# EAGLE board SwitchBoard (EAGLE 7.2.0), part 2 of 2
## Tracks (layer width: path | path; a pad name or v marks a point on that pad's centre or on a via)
5VIN  (via drill 0.4)
  Top 0.254: LED1.A 0.63,71.53 0.63,71.12 0.82,70.93 0.89,70.87 1.02,70.74 4.95,70.74 v5.08,70.87
  Top 0.406: X1.VBUS 6.32,78.77 JP1.1 8.57,78.74 C1.1 U1.4 | 0.63,71.53 LED1.A
  Bottom 0.406: 7.3,73.98 6.98,73.66 6.35,73.03 | 7.3,73.98 8.25,74.93 8.25,77.47 7.62,78.1 | 7.62,78.1 | 7.62,78.1 6.98,78.74 JP1.1 | v5.08,70.87 5.46,70.87 5.71,71.12 5.71,72.39 7.3,73.98
+5V  (via drill 0.6)
  Top 0.406: C21.1 C20.1 13.65,62.87 12.7,62.87 12.06,62.23 12.06,58.42 11.43,57.78 6.98,57.78 6.35,57.15 X2.9 | C21.1 | U12.1 18.41,62.23 17.46,63.18 C21.1 | U15.1 | U15.1 18.41,48.26 17.46,49.21 C26.1 C27.1 12.38,49.21 v12.06,49.53 | X2.9
  Bottom 0.406: v12.06,49.53 12.06,53.98 11.75,54.29 | 11.75,54.29 11.43,54.61 | 11.12,54.91 11.43,54.61 | 11.43,54.61 11.75,54.29 | X2.9 11.12,54.91 | 11.12,54.91 11.43,54.61
AGND  (via drill 0.4, 0.5, 0.6)
  Top 0.254: U12.9 U12.10 | U4.EXP v30.61,79.5 | 29.52,78.41 v29.08,77.98 | C15.- 41.31,86.96 U8.EXP 41.27,87.63 40.66,88.25 U8.7 | LED2.C 0.86,69.94 1.08,70.17 4.13,70.17 4.45,69.85 5.71,69.85 6.35,70.49 v6.98,70.49
  Top 0.406: v59.05,32.38 59.33,32.11 U5.21 | v55.88,29.21 55.88,28.58 55.88,27.94 57.15,26.67 57.78,26.67 58.42,26.04 59.05,25.4 59.33,25.12 U5.4 59.33,17.82 C7.1 59.05,17.46 v59.05,15.88 59.05,8.89 59.05,8.25 64.14,3.17 65.41,3.17 | v64.14,79.38 64.14,76.84 59.69,72.39 59.69,67.03 59.33,66.68 59.33,64.41 v59.05,64.13 59.33,63.85 U2.21 59.33,58.77 59.33,55.52 U2.4 59.37,54.3 C8.1 60,50.16 61.59,50.16 v62.23,49.53 | U7.4 141.96,22.58 v142.24,22.86 142.56,23.18 C13.1 | C17.1 142.56,51.12 v142.24,50.8 141.96,50.52 141.96,49.89 U10.4 141.96,46.71 141.96,44.73 U10.21 141.96,39.01 v141.96,38.38 141.96,34.92 143.51,33.38 143.51,30.48 144.15,29.84 148.59,29.84 156.21,37.46 156.21,45.72 157.48,46.99 157.81,47.32 160.35,47.32 X3.6 164.77,47.32 165.74,46.35 165.74,35.56 163.83,33.66 | U13.4 141.96,75.92 v142.24,76.2 142.24,77.78 C23.1 | U13.21 U13.20 U13.19 140.67,69.55 v141.6,70.49 | U13.16 U13.15 138.05,67.06 v138.43,66.68 | v141.6,16.51 141.96,16.15 U7.21 141.96,10.16 141.96,7.98 137.16,3.17 136.53,3.17 134.34,3.17 133.99,3.17 130.81,3.17 66.04,3.17 65.41,3.17 | U15.15 31.43,46.99 C24.2 C25.2 34.61,46.99 35.25,47.62 v36.2,47.62 | 27.94,46.99 27.3,46.35 27.3,41.27 27.94,40.64 U15.10 U15.9 | 27.94,46.99 U15.15 | U15.15 | U12.10 27.94,54.61 27.3,55.24 27.3,60.32 27.94,60.96 | 27.94,60.96 U12.15 31.43,60.96 C19.2 C18.2 35.25,61.28 35.56,61.28 v35.88,61.28 | U15.15 27.94,46.99 | 27.94,46.99 27.3,47.62 27.3,52.7 27.94,53.34 U12.9 | 163.83,33.66 | 163.83,33.66 JP5.1 | X1.GND 6.32,76.17 JP1.2 8.57,76.2 C1.2 8.89,75.56 9.52,74.93 9.52,73.66 10.16,73.03 12.7,73.03 13.02,73.34
  Top 0.406: U15.9 32.38,39.37 33.34,39.37 R24.1 | U4.7 U4.6 | U4.6 U4.5 | U4.6 28.17,78.74 U4.EXP | U4.EXP v30.61,77.98 30.82,77.76 U4.13 32.09,77.76 32.38,77.47 32.38,76.84 33.02,76.2 33.97,76.2 R10.1 33.97,75.56 R5.1 | U4.10 29.52,78.41 U4.EXP | C3.2 C4.2 24.45,78.74 | R11.2 2.22,87.95 1.9,87.63 1.49,87.22 0.86,86.58 LED4.C 0.86,83.6 1.27,83.19 1.9,83.19 3.17,83.19 v4.45,81.28 8.89,81.28 9.52,81.28 10.16,81.91 10.79,82.55 JP2.2 | JP2.2 10.79,84.29 JP3.1 | 13.02,73.34 R3.1 13.02,73.34 | U1.2 14.92,77.47 C2.2 | C9.2 C11.2 37.47,84.46 39.37,82.55 C15.- 39.37,80.6 39.37,79.38 | 27.94,60.96 27.3,61.6 27.3,62.87 33.97,69.53 R5.1 | 39.37,79.34 39.37,79.38 | 65.41,3.17 64.77,3.17 | R23.1 37.15,42.55 v35.56,42.55 | U15.9 29.46,40.01 v30.48,40.01 30.48,33.66 25.4,28.58 JP6.2 | 39.37,79.38 39.37,76.84 36.2,73.66 R5.1 | 13.33,95.25 10.79,92.71 JP2.2
  Bottom 0.254: v6.98,70.49 8.25,70.49 8.89,71.12 8.89,73.66 9.52,74.29 9.52,79.38 7.62,81.28 v4.45,81.28
  Bottom 0.406: v59.05,64.13 59.33,64.41 U3.21 59.33,70.49 | 59.33,70.49 59.33,70.76 | C6.1 59.33,79.97 U3.4 59.33,72.75 59.33,70.49 | v55.88,29.21 v59.05,32.38 59.33,32.66 U6.21 59.33,37.74 59.33,39.02 59.33,39.73 v59.05,40.01 59.33,40.28 U6.4 59.33,46 59.69,46.35 60.33,46.99 60.96,46.99 | 60.96,82.55 62.86,80.65 63.5,80.01 v64.14,79.38 | C17.1 142.88,52.39 142.88,51.44 v142.24,50.8 141.96,51.08 U11.4 141.96,58.06 141.96,60.04 U11.21 141.96,65.69 141.6,66.04 | v142.24,76.2 142.24,77.78 C23.1 | 142.08,78.58 141.96,78.71 U14.4 141.96,84.74 140.97,85.72 140.34,86.36 | 142.08,78.58 C23.1 | v141.96,38.38 141.96,37.19 U9.21 141.96,32.1 141.96,30.12 U9.4 141.96,27.59 141.96,25.37 C13.1 142.24,24.45 v142.24,22.86 140.97,21.59 140.97,17.14 v141.6,16.51 | U14.15 U14.16 138.71,86.72 139.06,86.36 140.34,86.36 | 140.34,86.36 140.66,86.69 U14.19 U14.20 U14.21 | 141.6,66.04 139.7,66.04 139.06,66.04 v138.43,66.68 | 141.6,66.04 v141.6,70.49 140.34,71.75 140.34,73.66 140.34,76.84 142.08,78.58 | v4.45,81.28 4.45,78.1 JP1.2 | v30.48,40.01 33.02,42.55 34.92,42.55 v35.56,42.55 35.56,46.35 36.2,46.99 v36.2,47.62 | C23.1 | C23.1 | 60.96,46.99 61.59,46.99 62.23,47.62 v62.23,49.53 | C8.1 59.37,48.58 60.96,46.99 | v35.88,61.28 37.14,61.28 40.64,57.78 40.64,53.98 40.64,52.7 41.27,52.07 JP7.3 | JP7.3
  other vias: 29.08,79.5 29.84,78.74 26.04,81.91 41.27,89.53 41.27,84.46 19.05,95.25 46.99,87 48.26,85.72 48.89,83.82 48.89,80.01 48.89,78.1 27.3,80.01 26.04,78.74 156.84,45.72 155.58,48.9 153.03,45.72 151.13,52.7 151.13,55.88 50.17,65.41 55.25,69.22 52.39,80.96 50.8,83.19 52.7,83.19 71.12,17.78 71.12,12.7 71.12,5.08 46.99,80.01 45.09,80.01 33.66,89.53 31.75,89.53 31.75,91.44 31.75,93.34 31.75,95.25 19.05,93.34 19.05,91.44 19.05,89.53 38.1,81.28 36.83,81.28 34.92,82.55 71.12,15.24 68.58,17.78 65.41,17.78 62.23,17.78 71.12,46.99 71.12,49.53 67.31,49.53 67.31,46.99 64.14,46.99 64.14,49.53 66.67,79.38 68.58,79.38 71.12,79.38 71.12,81.28 71.12,83.19 71.12,85.09 133.35,67.31 130.81,67.31 130.81,70.49 133.35,70.49 133.35,73.66 130.81,73.66 133.35,81.28 130.81,81.28 130.81,83.82 133.35,83.82 130.81,5.08 136.53,10.16 138.43,10.16 142.88,10.16 20.32,85.09 20.32,83.19 19.05,81.91 71.12,93.34 71.12,96.52 130.81,95.88 1.27,30.48 1.27,1.27 27.81,51.69 30.48,54.74 33.02,54.74 33.15,51.18 29.59,50.93 27.81,49.91 28.7,38.1 27.56,36.07 26.42,34.29
  pour Top (no thermals): 27.3,55.24 32.38,55.24 32.38,52.7 27.3,52.7
  pour Top (no thermals): 27.3,41.27 31.75,41.27 31.75,38.73 27.3,38.73
  pour Top (isolate 0.305, no thermals): 40.64,85.72 40.64,83.19 41.91,83.19 41.91,85.72
  pour Top (no thermals): 41.91,88.26 41.91,90.17 40.64,90.17 40.64,88.26
  pour Top (no thermals): 26.42,78.3 28.96,78.3 28.96,79.88 28.26,79.88 28.26,81.03 27.3,81.91 27.3,87 24.13,87 24.13,82.55 25.4,82.55 25.4,79.38 20.95,79.38 20.95,78.1 26.04,78.1
  pour Bottom (isolate 0.305, no thermals): 20.32,69.22 20.32,87 38.73,87 38.73,69.22
  pour Top (isolate 0.305, no thermals): 37.47,85.09 41.27,85.09 41.27,82.55 38.73,82.55 37.47,83.82
  pour Bottom (isolate 0.305, rank 6): -3.81,67.94 -3.81,102.87 -3.18,103.5 172.09,103.5 172.09,-2.54 -3.81,-2.54 -4.45,-1.91 -4.45,33.02 -3.18,33.02 -0.64,32.38 22.23,32.38 22.86,33.02 22.86,34.29 26.04,37.46 26.04,63.5 25.4,64.13 24.13,67.94
  pour Top (isolate 0.305, rank 6): -7.62,32.38 -11.43,-3.81 175.26,-3.81 173.99,104.78 -8.25,105.41 -6.35,67.94 24.13,67.94 26.04,63.5 26.04,38.1 22.23,32.38
CHRG
  Top 0.406: R1.2 LED1.C
DIN+  (via drill 0.6)
  Top 0.406: U2.3 58.67,56.26 56.52,58.42 55.88,58.42 55.25,57.78 55.25,55.24 v54.61,54.61 | U12.13 v36.83,58.42 37.47,59.05 48.26,59.05 49.53,59.05 | 49.53,59.05 v50.17,59.69 49.53,59.05
  Bottom 0.406: v36.83,58.42 37.47,58.42 39.37,56.52 39.37,48.9 41.27,46.99 JP7.7 | JP7.7 | JP7.7 | v54.61,54.61 53.97,54.61 53.34,55.24 53.34,55.88 53.97,56.52 53.97,57.78 53.34,58.42 51.44,58.42 v50.17,59.69
DIN+2  (via drill 0.5)
  Top 0.406: U2.22 58.67,58.67 v58.42,58.42 | v53.97,49.53 53.97,46.99 53.34,46.35 53.34,33.02 v53.97,32.38 | U5.3 58.67,24.51 57.78,25.4 v57.15,25.4
  Bottom 0.406: v57.15,25.4 55.88,26.67 53.97,28.58 v53.97,32.38 | v53.97,49.53 53.97,50.8 55.25,52.07 57.15,53.98 | v58.42,58.42 58.42,55.24 57.15,53.98 | 57.15,53.98 55.25,55.88 55.25,57.47 55.25,58.74 R6.1
DIN+3  (via drill 0.5)
  Top 0.406: U5.22 58.67,27.05 v60.33,25.4 | U7.3 142.62,19.43 v142.24,19.05
  Bottom 0.406: v60.33,25.4 60.33,24.13 | R12.1 55.56,22.54 57.15,24.13 60.33,24.13 | 67.94,2.54 78.11,2.54 130.81,2.54 131.44,2.54 132.08,2.54 138.43,2.54 140.97,5.08 140.97,11.43 140.97,13.97 142.88,15.88 142.88,16.51 142.88,17.78 142.24,18.41 v142.24,19.05 | 67.94,2.54 67.31,2.54 | 60.33,24.13 60.33,20.95 60.33,6.98 63.5,3.81 64.77,2.54 67.94,2.54
DIN+4  (via drill 0.5)
  Top 0.406: U7.22 142.62,12.32 143.19,11.75 R17.1 149.54,11.75 150.18,11.75 v151.13,12.7 | U10.3 142.62,46.61 142.88,46.35 143.51,46.35 146.05,46.35 146.69,45.72 v146.69,43.81
  Bottom 0.406: v151.13,12.7 151.13,41.91 149.86,43.18 147.96,43.18 147.32,43.18 v146.69,43.81
DIN+5
  Top 0.406: 147.63,39.37 R19.1 | R19.1 150.18,39.69 151.13,40.64 151.77,41.27 151.77,46.35 152.4,46.99 152.4,71.12 151.77,71.75 151.13,72.39 150.5,73.03 149.86,73.03 142.88,73.03 142.62,73.28 U13.3 | U10.22 142.62,44.2 142.88,44.45 144.15,44.45 144.78,43.81 144.78,43.18 146.05,41.91 146.05,40.64 146.69,40.01 147.64,40.01 R19.1
DIN+_DCHN  (via drill 0.6)
  Top 0.406: JP7.8 45.09,47.62 v47.62,47.62
  Bottom 0.406: X6.3 10.16,15.88 | v47.62,47.62 47.62,46.35 47.62,45.72 47.62,42.55 47.62,41.91 48.26,41.27 48.26,29.21 48.26,28.58 47.62,27.94 36.83,27.94 36.2,27.94 27.94,19.68 15.88,19.68 12.06,15.88 X6.3 | X6.3
DIN+_IN
  Top 0.406: U12.4 16.51,58.42 X2.3
DIN-  (via drill 0.5, 0.6)
  Top 0.406: U12.12 v35.56,57.15 37.47,57.15 38.42,58.1 | 38.42,58.1 38.73,58.42 | v53.34,76.2 52.7,75.56 52.7,73.66 52.07,73.03 50.17,73.03 49.53,72.39 49.53,70.49 49.53,69.85 50.17,69.22 51.44,67.94 51.44,59.05 50.8,58.42 38.73,58.42 | 38.73,58.42 38.42,58.1
  Bottom 0.406: U3.3 58.67,73.28 58.42,73.03 57.15,73.03 56.52,73.66 56.52,75.56 55.88,76.2 v53.34,76.2 | v35.56,57.15 37.47,57.15 38.73,55.88 38.73,50.8 38.73,48.26 41.91,45.09 JP7.9 | JP7.9
DIN-2  (via drill 0.5, 0.6)
  Top 0.406: v60.96,48.9 60.96,48.26 60.33,47.62 59.05,47.62 v58.42,47.62
  Bottom 0.406: 54.93,72.39 R7.1 54.92,72.71 55.25,72.39 58.42,72.39 58.67,72.14 U3.22 58.67,65.66 57.78,64.77 57.78,62.23 60.96,59.05 v60.96,48.9 | U6.3 58.67,45.09 58.67,47.37 v58.42,47.62
DIN-3  (via drill 0.5)
  Top 0.406: v51.44,38.1 51.44,20.95 51.44,20.32 53.97,17.78 53.97,8.25 61.59,0.63 62.23,0.63 64.77,0.63 134.62,0.63 142.88,0.63 | v148.59,13.97 151.77,13.97 152.4,13.34 152.4,8.89 144.15,0.63 142.88,0.63 | 143.51,0.63 142.88,0.63
  Bottom 0.406: U6.22 58.67,38.48 58.42,38.73 58.1,39.05 55.56,39.05 R13.1 52.39,39.05 v51.44,38.1 | U9.3 142.62,29.59 142.62,31.5 143.51,32.38 144.15,32.38 147.32,32.38 147.96,31.75 147.96,30.48 147.96,22.86 147.32,22.23 147.32,15.88 147.32,15.24 v148.59,13.97
DIN-4
  Bottom 0.406: U9.22 142.62,35.94 142.62,37.21 142.88,37.46 147.64,37.46 R18.1 147.96,39.37 146.69,40.64 145.42,41.91 144.78,42.55 144.15,43.18 144.15,45.72 148.59,50.16 148.59,50.8 148.59,53.98 148.59,56.52 147.32,57.78 146.05,59.05 142.88,59.05 142.62,58.8 142.62,57.53 U11.3
DIN-5
  Bottom 0.406: U14.3 142.62,83.57 142.88,83.82 144.78,83.82 148.59,80.01 148.59,76.2 147.96,75.56 | U11.22 142.62,63.88 142.88,64.13 146.05,64.13 146.69,64.77 147.64,64.77 R20.1 149.55,65.09 149.86,65.41 149.86,67.94 147.96,69.85 147.96,71.75 147.96,75.56 | 147.96,75.56
DIN-_DCHN  (via drill 0.6)
  Top 0.406: X6.7 11.43,14.5 12.06,15.14 v12.06,20.95
  Bottom 0.406: JP7.10 45.09,44.45 45.72,43.81 45.72,40.64 45.72,40.01 46.36,39.37 46.36,31.75 46.36,31.12 46.36,30.48 45.72,29.84 34.29,29.84 33.66,29.21 26.04,21.59 12.7,21.59 v12.06,20.95 | JP7.10
DIN-_IN
  Top 0.406: U12.5 16.51,57.15 10.16,50.8 10.16,49.53 10.06,49.43 X2.7
DOUT+  (via drill 0.6)
  Top 0.406: 147.64,66.68 R21.1 | U13.22 142.62,67.56 142.88,67.31 144.15,67.31 144.78,67.94 146.69,67.94 147.64,66.99 R21.1 | R21.1 147.96,62.23 v148.59,61.6 | X3.3 160.02,51.44 | 160.02,51.44 159.39,51.44 | v156.84,57.15 158.12,57.15 158.75,56.52 158.75,52.7 158.75,52.07 159.39,51.44 | 159.39,51.44 160.02,51.44
  Bottom 0.406: v148.59,61.6 151.13,61.6 155.58,57.15 v156.84,57.15
DOUT-  (via drill 0.6)
  Top 0.406: 154.31,62.87 154.31,52.7 156.95,50.06 X3.7 | 154.31,62.87 v154.31,64.13 154.31,62.87
  Bottom 0.406: 142.62,88.9 U14.22 142.62,88.9 | v154.31,64.13 153.03,65.41 153.03,69.85 151.77,71.12 151.77,80.65 146.05,86.36 R22.1 145.09,88.59 144.78,88.9 144.15,89.53 143.26,89.53 142.62,88.9
GND  (via drill 0.4)
  Top 0.406: C20.2 C21.2 16.51,60.96 U12.2 20.32,60.96 20.95,60.32 20.95,55.24 20.32,54.61 U12.7 | C20.2 | U12.8 20.32,53.34 20.95,52.7 20.95,47.62 20.32,46.99 | 20.32,46.99 20.95,46.35 20.95,41.27 20.32,40.64 U15.7 U15.8 | 20.32,46.99 | 20.32,46.99 U15.2 16.83,46.99 C26.2 C27.2 13.65,47.62 12.06,47.62 11.75,47.31 11.13,46.69 X2.6
  other vias: 19.56,65.66 0.89,65.79 18.8,50.93 20.7,50.93 18.54,35.94 0.89,35.81
  pour Top (no thermals): 20.95,55.24 20.95,52.7 15.88,52.7 15.88,55.24
  pour Top (no thermals): 20.95,41.27 20.95,38.73 15.88,38.73 15.88,41.27
  pour Top: -5.71,67.31 20.95,67.31 22.86,63.5 22.86,38.73 19.68,34.29 -6.35,34.29
  pour Bottom (isolate 0.305): -4.45,67.31 21.59,67.31 24.13,62.23 23.49,38.73 20.32,33.66 -3.81,33.66 -4.45,65.41
GND_DCHN
  Top 0.406: X6.6 13.66,11.76 14.61,12.7 14.61,20.95 15.24,21.59 26.04,21.59 34.29,29.84 45.72,29.84 46.36,30.48 46.36,44.45 46.36,45.09 45.72,45.72 43.81,45.72 43.18,46.35 43.18,51.44 43.81,52.07 JP7.4
IN+  (via drill 0.5, 0.6)
  Top 0.406: U2.19 60.63,58.75 v62.23,57.15 | U2.13 64.54,58.83 62.86,57.15 | U2.15 63.25,58.8 62.86,58.42 62.86,57.78 v62.23,57.15 | U2.17 61.93,58.72 62.23,58.42 v62.23,57.15 | U2.6 60.63,55.55 v62.23,57.15 | U2.8 61.93,55.58 62.23,55.88 v62.23,57.15 | U2.12 64.54,55.47 62.86,57.15 | U2.10 63.25,55.5 62.86,55.88 62.86,56.52 v62.23,57.15 | 62.86,57.15 v62.23,57.15 | U5.6 60.63,23.8 v62.23,25.4 | U5.8 61.92,23.82 62.23,24.13 v62.23,25.4 | U5.10 63.25,23.75 62.86,24.13 62.86,24.77 v62.23,25.4 | U5.12 64.54,23.72 62.86,25.4 | U5.19 60.63,27 v62.23,25.4 | U5.17 61.92,26.98 62.23,26.67 v62.23,25.4 | U5.15 63.25,27.05 62.86,26.67 62.86,26.04 v62.23,25.4 | U5.13 64.54,27.08 62.86,25.4 | 62.86,25.4 v62.23,25.4 | U7.19 140.67,16.81 139.7,17.78 | U7.17 139.37,16.84 139.37,17.48 139.06,17.78 | U7.13 136.75,16.74 136.75,17.55 136.53,17.78 | U7.15 138.05,16.76 138.05,17.53 137.8,17.78 | U7.12 136.75,18.82 136.75,18.01 136.53,17.78 | U7.10 138.05,19.43 138.05,18.03 137.8,17.78 | 139.37,19.36 U7.8 139.37,18.09 139.06,17.78 | 139.06,17.78 137.8,17.78 | 137.8,17.78 136.53,17.78 | 136.53,17.78 v135.89,17.78 | 139.7,17.78 139.06,17.78 | U7.6 140.67,18.75 139.7,17.78 | 137.8,17.78 139.06,17.78 | 138.43,17.78 139.06,17.78 | v139.7,45.72 140.67,46.69 U10.6 | U10.19 140.67,44.75 v139.7,45.72 | U10.17 139.37,45.39 v139.7,45.72 | U10.8 139.37,46.05 v139.7,45.72 | U10.10 138.05,47.37 v139.7,45.72 | U10.12 136.75,46.76 137.8,45.72 | 137.8,45.72 v139.7,45.72 | U10.13 136.75,44.68 137.8,45.72 | U10.15 138.05,44.07 v139.7,45.72 | U13.13 136.75,70.71 137.8,71.75 | U13.12 136.75,72.8 137.8,71.75 | U13.10 138.05,72.77 v139.06,71.75 | 137.8,71.75 v139.06,71.75
  Top 0.406: U13.6 140.67,72.72 139.7,71.75 v139.06,71.75 | U13.8 139.37,72.06 v139.06,71.75
  Bottom 0.406: 72.39,24.77 73.03,25.4 73.03,36.2 73.03,47.62 | 72.39,24.77 66.04,24.77 65.41,25.4 v62.23,25.4 | v135.89,17.78 134.62,16.51 129.54,16.51 | v139.7,45.72 137.16,45.72 136.53,45.72 135.89,45.72 133.99,43.81 130.81,43.81 129.54,43.81 | v139.06,71.75 132.08,71.75 129.54,71.75 | 128.91,67.94 128.91,60.96 128.91,57.15 128.91,55.88 128.91,44.45 129.54,43.81 | 128.91,67.94 128.91,68.58 | v62.23,57.15 64.14,57.15 65.41,57.15 66.67,55.88 72.39,55.88 | 129.54,16.51 128.91,15.88 128.91,4.45 128.27,3.81 74.3,3.81 73.66,3.81 73.03,4.45 73.03,5.08 73.03,8.89 73.03,24.13 72.39,24.77 | 129.54,16.51 128.91,17.14 128.91,35.56 128.91,38.1 128.91,41.91 128.91,43.18 129.54,43.81 | 73.03,48.26 73.03,47.62 | 73.03,47.62 73.03,51.44 73.03,55.24 72.39,55.88 | 128.91,92.71 127,94.62 74.93,94.62 73.03,92.71 73.03,81.91 73.03,56.52 72.39,55.88 | 128.91,92.71 128.91,72.39 129.54,71.75 | 128.91,68.58 128.91,67.94 | 128.91,68.58 128.91,71.12 129.54,71.75 | 130.81,94.62 128.91,92.71 | 130.81,94.62 | 130.81,94.62 150.39,94.62 arc-45 150.57,94.54 JP8.1
  pour Top (no thermals): 60.33,58.42 65.41,58.42 65.41,55.88 60.33,55.88
  pour Top (no thermals): 61.28,26.67 65.41,26.67 65.41,24.13 61.28,24.13
  pour Top (no thermals): 135.89,19.05 140.72,19.05 140.72,16.51 135.89,16.51
  pour Top (no thermals): 135.89,46.99 140.97,46.99 140.97,44.45 135.89,44.45
  pour Top (no thermals): 136.53,70.49 136.53,73.03 140.34,73.03 140.34,72.01 138.81,70.49
IN-  (via drill 0.5, 0.6)
  Top 0.406: v139.06,31.12 132.08,31.12 129.54,31.12 v127.63,31.12 | v136.53,59.05 v127.63,59.05 | v62.23,39.37 v74.3,39.37 | v64.77,71.75 v74.3,71.75 | v136.53,85.09 v127.63,85.09 127.63,90.17 130.81,93.34 146.58,93.34 arc-45 146.76,93.27 154.94,85.09 154.94,83.19 JP9.1
  Bottom 0.406: U9.13 136.75,33.02 136.75,32.16 137.16,31.75 137.8,31.12 | U9.12 136.75,30.07 137.8,31.12 | U9.15 138.05,32.13 v139.06,31.12 | U9.10 138.05,30.1 v139.06,31.12 | U9.8 139.37,30.81 v139.06,31.12 | U9.17 139.37,31.42 v139.06,31.12 | U9.19 140.66,32.08 139.7,31.12 | 139.7,31.12 v139.06,31.12 | U9.6 140.66,30.15 139.7,31.12 | 137.8,31.12 v139.06,31.12 | v62.23,39.37 60.63,37.77 U6.19 | U6.12 64.54,40.41 63.5,39.37 | 63.5,39.37 v62.23,39.37 | U6.13 64.54,38.33 63.5,39.37 | U6.17 61.93,39.07 v62.23,39.37 | U6.8 61.93,39.67 v62.23,39.37 | U6.15 63.25,38.35 v62.23,39.37 | U6.10 63.25,40.39 v62.23,39.37 | U3.6 60.63,72.72 61.59,71.75 | 61.59,71.75 62.23,71.75 | U3.19 60.63,70.79 61.59,71.75 | U3.8 61.93,72.06 62.23,71.75 | U3.17 61.93,71.45 62.23,71.75 | U3.10 63.25,72.14 62.86,71.75 | 62.86,71.75 62.23,71.75 | U3.15 63.25,71.37 62.86,71.75 | U3.12 64.54,72.16 64.14,71.75 | 64.14,71.75 62.23,71.75 | U3.13 64.54,71.35 64.14,71.75 | 139.06,59.05 139.7,59.05 | 139.7,59.05 140.34,59.69 140.66,60.02 U11.19 | U11.6 140.66,58.09 139.7,59.05 | U11.8 139.37,58.75 139.06,59.05 | U11.17 139.37,59.36 139.06,59.05 | U11.15 138.05,60.07 139.06,59.05 | U11.10 138.05,58.04 139.06,59.05 | U11.13 136.75,59.46 137.16,59.05 | 137.16,59.05 139.06,59.05 | U11.12 136.75,58.65 137.16,59.05 | U14.6 140.66,84.76 140.34,85.09 139.06,85.09 | U14.8 139.37,84.79 139.06,85.09 | U14.10 138.05,84.71 138.43,85.09 139.06,85.09 | U14.12 136.75,84.68 137.16,85.09 | U14.13 136.75,85.5 137.16,85.09 | 137.16,85.09 139.06,85.09 | U6.6 60.63,40.97 v62.23,39.37 | 127.63,58.42 127.63,57.78 v127.63,31.12 127.63,5.71 127,5.08 74.93,5.08 74.3,5.71 v74.3,39.37 74.3,41.27 74.3,50.16
  Bottom 0.406: 127.63,58.42 v127.63,59.05 | v127.63,59.05 127.63,68.58 | 127.63,68.58 127.63,69.22 | v136.53,85.09 137.16,85.09 | 137.16,59.05 v136.53,59.05 | 62.23,71.75 v64.77,71.75 | v127.63,59.05 127.63,58.42 | 74.3,50.8 74.3,50.16 | 74.3,50.16 v74.3,71.75 | v74.3,71.75 74.3,72.39 | v74.3,71.75 74.3,72.39 | 74.3,72.39 74.3,82.55 74.3,85.09 74.3,92.07 75.56,93.34 126.36,93.34 127.63,92.07 127.63,85.72 | 127.63,85.72 v127.63,85.09 | v127.63,85.09 127.63,69.22 | 127.63,69.22 127.63,68.58 | v127.63,85.09 127.63,85.72
  pour Bottom: 60.33,73.03 65.41,73.03 65.41,70.49 60.33,70.49
  pour Bottom (isolate 0.305, no thermals): 60.33,40.64 65.41,40.64 65.41,38.1 60.33,38.1
  pour Bottom (no thermals): 140.97,32.38 140.97,29.84 135.89,29.84 135.89,32.38
  pour Bottom (no thermals): 135.89,60.32 140.97,60.32 140.97,57.78 135.89,57.78
  pour Bottom (no thermals): 137.8,86.36 139.06,85.09 140.34,85.09 140.34,83.82 136.53,83.82 136.53,86.36
LB_REF
  Top 0.406: R5.2 R4.1 28.87,73.68 U4.9
LBO  (via drill 0.6)
  Top 0.406: v31.75,75.56 30.82,76.5 U4.12 | v31.12,71.12 30.8,70.8 28.25,70.8 R14.1
  Bottom 0.406: v31.75,75.56 31.75,71.75 v31.12,71.12
N$1  (via drill 3)
  other vias: 2.54,94.62
N$3
  Top 0.254: U8.5 44.88,87.75 C14.1 45.09,87.63 44.2,86.75 U8.3
  pour Top (no thermals): 43.56,87.76 44.89,87.76 44.77,87.25 44.2,86.74 43.56,86.74
N$4
  Top 0.254: 44.77,89.53 C14.2 44.77,89.53 | U8.6 43.16,88.25 43.81,88.9 44.45,89.53 44.77,89.53
N$5
  Top 0.254: LED2.A 6.98,69.22 8.25,69.22 8.7,69.66 R2.2
N$6
  Top 0.406: R8.1 37.47,80.01 37.78,79.69 R9.2
N$7
  Top 0.406: LED3.C 5.39,90.17 R11.1
N$8  (via drill 0.6)
  Top 0.406: T1.C v17.14,72.39 | v8.25,82.55 7.62,83.19 7.62,83.5 R16.1
  Bottom 0.406: v17.14,72.39 15.88,73.66 15.88,74.93 15.88,76.2 15.88,78.74 13.97,80.65 13.33,81.28 9.52,81.28 v8.25,82.55
N$9
  Top 0.406: LED4.A R16.2
N$10
  Bottom 0.406: JP5.2 160.66,37.64 X3.G1 164.64,38.91 165.1,39.37 165.74,40.01 165.74,62.87 165.1,63.5 164.64,63.96 X3.G2
N$11
  Top 0.406: T1.B R15.1 23.81,71.12 R14.2
N$12
  Bottom 0.406: X6.G1 2.36,3.35 1.9,3.81 1.9,4.45 1.9,27.94 2.36,28.4 X6.G2 13.16,28.4 JP6.1
N$13  (via drill 3)
  other vias: 167.01,94.62
N$14  (via drill 3)
  other vias: 167.01,2.54
N$15  (via drill 3)
  other vias: 15.24,3.17
OUT_1  (via drill 0.5, 0.6)
  Top 0.406: v76.12,57.15 v70.48,57.15 70.48,51.44 69.85,50.8 60.96,50.8 60.33,51.44 60.33,52.7 60,53.03 U2.5
  Bottom 0.254: X4.1 v76.12,57.15
  Bottom 0.406: X4.1 X5.1 | U3.5 60,77.78 60.33,78.1 69.85,78.1 70.48,77.47 v70.48,57.15
OUT_2  (via drill 0.5, 0.6)
  Top 0.406: v78.89,58.41 76.83,58.42 v69.22,58.42 69.22,52.07 68.58,51.44 61.59,51.44 61.29,51.74 U2.7
  Bottom 0.254: X4.2 v78.89,58.41
  Bottom 0.406: X4.2 X5.2 | U3.7 61.29,77.17 61.59,77.47 68.58,77.47 69.22,76.84 v69.22,58.42
OUT_3  (via drill 0.5, 0.6)
  Top 0.406: U2.9 62.59,52.35 62.86,52.07 67.31,52.07 67.94,52.7 v67.94,59.69 v81.64,59.69
  Bottom 0.254: X4.3 v81.64,59.69
  Bottom 0.406: X4.3 X5.3 | U3.9 62.59,76.56 62.86,76.84 67.31,76.84 67.94,76.2 v67.94,59.69
OUT_4  (via drill 0.5, 0.6)
  Top 0.406: U2.11 63.88,52.96 64.14,52.7 66.04,52.7 66.67,53.34 v66.67,60.96 v84.4,60.96
  Bottom 0.254: X4.4 v84.4,60.96
  Bottom 0.406: X4.4 X5.4 | U3.11 63.88,75.95 64.14,76.2 66.04,76.2 66.67,75.56 v66.67,60.96
OUT_5  (via drill 0.5, 0.6)
  Top 0.406: U2.14 63.88,61.34 64.14,61.6 v64.14,62.23 v87.17,62.23
  Bottom 0.254: X4.5 v87.17,62.23
  Bottom 0.406: X4.5 X5.5 | U3.14 63.88,67.56 64.14,67.31 v64.14,62.23
OUT_6  (via drill 0.5, 0.6)
  Top 0.406: U2.16 62.59,61.95 62.86,62.23 v62.86,63.5 v89.92,63.5
  Bottom 0.254: X4.6 v89.92,63.5
  Bottom 0.406: X4.6 X5.6 | U3.16 62.59,67.59 62.86,67.31 v62.86,63.5
OUT_7  (via drill 0.5, 0.6)
  Top 0.406: U2.18 61.29,62.56 61.59,62.87 v61.59,64.77 v92.69,64.77
  Bottom 0.254: X4.7 v92.69,64.77
  Bottom 0.406: X5.7 X4.7 | U3.18 61.29,67.61 61.59,67.31 v61.59,64.77
OUT_8  (via drill 0.5, 0.6)
  Top 0.406: v95.45,66.04 v60.33,66.04 60.33,63.5 60,63.17 U2.20
  Bottom 0.254: X4.8 v95.45,66.04
  Bottom 0.406: X5.8 X4.8 | v60.33,66.04 60.33,66.68 60,67 U3.20
OUT_9  (via drill 0.5, 0.6)
  Top 0.406: v98.2,26.04 v70.48,26.04 70.48,19.68 69.85,19.05 60.33,19.05 59.99,19.38 U5.5
  Bottom 0.254: X4.9 v98.2,26.04
  Bottom 0.406: X5.9 X4.9 | U6.5 60,45.39 60.33,45.72 69.85,45.72 70.48,45.09 v70.48,26.04
OUT_10  (via drill 0.5, 0.6)
  Top 0.406: v100.96,27.3 v69.22,27.3 69.22,20.32 68.58,19.68 61.59,19.68 61.29,19.99 U5.7
  Bottom 0.254: X4.10 v100.96,27.3
  Bottom 0.406: X4.10 X5.10 | U6.7 61.29,44.78 61.59,45.09 68.58,45.09 69.22,44.45 v69.22,27.3
OUT_11  (via drill 0.5, 0.6)
  Top 0.406: v103.73,28.58 v67.94,28.58 67.94,20.95 67.31,20.32 62.86,20.32 62.58,20.6 U5.9
  Bottom 0.254: X4.11 v103.73,28.58
  Bottom 0.406: X4.11 X5.11 | U6.9 62.59,44.17 62.86,44.45 67.31,44.45 67.94,43.81 v67.94,28.58
OUT_12  (via drill 0.5, 0.6)
  Top 0.406: v106.48,29.84 v66.67,29.84 66.67,21.59 66.04,20.95 64.14,20.95 63.88,21.21 U5.11
  Bottom 0.254: X4.12 v106.48,29.84
  Bottom 0.406: X4.12 X5.12 | U6.11 63.88,43.56 64.14,43.81 66.04,43.81 66.67,43.18 v66.67,29.84
OUT_13  (via drill 0.5, 0.6)
  Top 0.406: v109.24,31.12 v64.14,31.12 64.14,29.84 63.88,29.59 U5.14
  Bottom 0.254: X4.13 v109.24,31.12
  Bottom 0.406: X4.13 X5.13 | U6.14 63.88,34.54 64.14,34.29 v64.14,31.12
OUT_14  (via drill 0.5, 0.6)
  Top 0.406: v112.01,32.38 v62.86,32.38 62.86,30.48 62.58,30.2 U5.16
  Bottom 0.254: X4.14 v112.01,32.38
  Bottom 0.406: X4.14 X5.14 | U6.16 62.59,34.57 62.86,34.29 v62.86,32.38
OUT_15  (via drill 0.5, 0.6)
  Top 0.406: v114.77,33.66 v61.59,33.66 61.59,31.75 61.29,31.45 U5.18
  Bottom 0.254: X4.15 v114.77,33.66
  Bottom 0.406: X4.15 X5.15 | U6.18 61.29,34.59 61.59,34.29 v61.59,33.66
OUT_16  (via drill 0.5, 0.6)
  Top 0.406: v117.52,34.92 73.66,34.92 v60.33,34.92 60.33,30.48 59.99,30.15 U5.20
  Bottom 0.254: X4.16 v117.52,34.92
  Bottom 0.406: X4.16 X5.16 | U6.20 60,35.26 v60.33,34.92
OUT_17  (via drill 0.5, 0.6)
  Top 0.406: U7.5 141.3,21.92 141.27,21.92 140.97,22.23 140.97,26.04 | v120.29,26.67 v140.97,26.67 140.97,26.04 | 140.97,24.77 140.97,26.04
  Bottom 0.406: X4.17 X5.17 v120.29,26.67 | U9.5 141.3,27 v140.97,26.67
OUT_18  (via drill 0.5, 0.6)
  Top 0.406: v123.04,25.4 v139.7,25.4 139.7,22.23 140,21.92 U7.7
  Bottom 0.254: X5.18 v123.04,25.4
  Bottom 0.406: X4.18 X5.18 | v139.7,25.4 139.7,26.67 140,26.97 U9.7
OUT_19  (via drill 0.5, 0.6)
  Top 0.406: v125.81,24.13 v138.43,24.13 138.43,22.23 138.71,21.95 U7.9
  Bottom 0.254: X5.19 v125.81,24.13
  Bottom 0.406: X4.19 X5.19 | v138.43,24.13 138.43,26.67 138.71,26.95 U9.9
OUT_20  (via drill 0.5, 0.6)
  Top 0.406: v77.5,22.86 v137.16,22.86 137.16,22.23 137.41,21.97 U7.11
  Bottom 0.254: X5.20 v77.5,22.86
  Bottom 0.406: X5.20 X4.20 | v137.16,22.86 137.16,26.67 137.41,26.92 U9.11
OUT_21  (via drill 0.5, 0.6)
  Top 0.406: v80.26,21.59 v134.62,21.59 134.62,13.97 135.25,13.34 137.16,13.34 137.41,13.59 U7.14
  Bottom 0.254: X5.21 v80.26,21.59
  Bottom 0.406: X5.21 X4.21 | U9.14 137.41,35.31 137.16,35.56 135.25,35.56 134.62,34.92 v134.62,21.59
OUT_22  (via drill 0.5, 0.6)
  Top 0.406: v83.01,20.32 v133.35,20.32 133.35,13.34 133.99,12.7 138.43,12.7 138.71,12.98 U7.16
  Bottom 0.254: X5.22 v83.01,20.32
  Bottom 0.406: X5.22 X4.22 | U9.16 138.71,35.92 138.43,36.2 133.99,36.2 133.35,35.56 v133.35,20.32
OUT_23  (via drill 0.5, 0.6)
  Top 0.406: v85.77,19.04 128.27,19.05 v132.08,19.05 132.08,12.7 132.72,12.07 139.7,12.07 140,12.37 U7.18
  Bottom 0.254: X5.23 v85.77,19.04
  Bottom 0.406: X5.23 X4.23 | U9.18 140,36.53 139.7,36.83 132.72,36.83 132.08,36.2 v132.08,19.05
OUT_24  (via drill 0.5, 0.6)
  Top 0.406: v88.55,17.78 v130.81,17.78 130.81,12.07 131.44,11.43 140.97,11.43 141.3,11.76 U7.20
  Bottom 0.254: X5.24 v88.55,17.78
  Bottom 0.406: X5.24 X4.24 | U9.20 141.3,37.13 140.97,37.46 131.44,37.46 130.81,36.83 v130.81,17.78
OUT_25  (via drill 0.5, 0.6)
  Top 0.406: v91.31,54.61 v140.97,54.61 140.97,50.16 141.3,49.83 U10.5
  Bottom 0.406: X4.25 X5.25 | X4.25 | X4.25 v91.31,54.61 | U11.5 141.3,54.94 v140.97,54.61
OUT_26  (via drill 0.5, 0.6)
  Top 0.406: v94.06,53.34 v139.7,53.34 139.7,50.8 140,50.49 U10.7
  Bottom 0.406: X5.26 X4.26 | X4.26 | X4.26 v94.06,53.34 | U11.7 140,53.64 v139.7,53.34
OUT_27  (via drill 0.5, 0.6)
  Top 0.406: v96.83,52.07 v138.43,52.07 138.43,50.16 138.71,49.88 U10.9
  Bottom 0.406: X4.27 X5.27 | X4.27 | X4.27 v96.83,52.07 | v138.43,52.07 138.43,54.61 138.71,54.89 U11.9
OUT_28  (via drill 0.5, 0.6)
  Top 0.406: v99.59,50.79 127,50.8 v137.16,50.8 137.41,50.55 U10.11
  Bottom 0.406: X5.28 X4.28 | X4.28 | X4.28 v99.59,50.79 | v137.16,50.8 137.16,53.98 137.41,54.23 U11.11
OUT_29  (via drill 0.5)
  Top 0.406: U10.14 137.41,41.53 137.16,41.27 135.25,41.27 134.62,41.91 v134.62,49.53 v102.34,49.53
  Bottom 0.254: X4.29 v102.34,49.53
  Bottom 0.406: X5.29 X4.29 | U11.14 137.41,63.25 137.16,63.5 135.25,63.5 134.62,62.87 v134.62,49.53
OUT_30  (via drill 0.5, 0.6)
  Top 0.406: v105.1,48.26 v133.35,48.26 133.35,41.27 133.99,40.64 138.43,40.64 138.71,40.92 U10.16
  Bottom 0.254: X4.30 v105.1,48.26
  Bottom 0.406: X5.30 X4.30 | U11.16 138.71,63.86 138.43,64.13 133.99,64.13 133.35,63.5 v133.35,48.26
OUT_31  (via drill 0.5, 0.6)
  Top 0.406: v107.87,46.99 v132.08,46.99 132.08,40.64 132.72,40.01 139.7,40.01 140,40.31 U10.18
  Bottom 0.254: X4.31 v107.87,46.99
  Bottom 0.406: X5.31 X4.31 | U11.18 140,64.47 139.7,64.77 132.72,64.77 132.08,64.13 v132.08,46.99
OUT_32  (via drill 0.5, 0.6)
  Top 0.406: v110.64,45.72 v130.81,45.72 130.81,40.01 131.44,39.37 140.97,39.37 141.3,39.7 U10.20
  Bottom 0.254: X4.32 v110.64,45.72
  Bottom 0.406: X5.32 X4.32 | U11.20 141.3,65.07 140.97,65.41 131.44,65.41 130.81,64.77 v130.81,45.72
OUT_33  (via drill 0.5, 0.6)
  Top 0.406: v113.39,80 v140.96,80 v140.97,80.01 140.97,76.2 141.3,75.87 U13.5
  Bottom 0.254: X4.33 v113.39,80
  Bottom 0.406: X5.33 X4.33 | v140.97,80.01 140.97,80.65 141.3,80.97 U14.5
OUT_34  (via drill 0.5, 0.6)
  Top 0.406: v116.15,78.74 v139.7,78.74 139.7,76.2 140,75.9 U13.7
  Bottom 0.254: X4.34 v116.15,78.74
  Bottom 0.406: X5.34 X4.34 | v139.7,78.74 139.7,80.65 140,80.95 U14.7
OUT_35  (via drill 0.5, 0.6)
  Top 0.406: v118.92,77.47 v138.43,77.47 138.43,76.2 138.71,75.92 U13.9
  Bottom 0.254: X4.35 v118.92,77.47
  Bottom 0.406: X5.35 X4.35 | v138.43,77.47 138.43,80.65 138.71,80.92 U14.9
OUT_36  (via drill 0.5, 0.6)
  Top 0.406: v121.66,76.19 121.67,76.2 v137.16,76.2 137.41,75.95 U13.11
  Bottom 0.254: X4.36 v121.66,76.19
  Bottom 0.406: X5.36 X4.36 | v137.16,76.2 137.16,80.65 137.41,80.9 U14.11
OUT_37  (via drill 0.5, 0.6)
  Top 0.406: U13.14 137.41,67.56 137.16,67.31 135.89,67.31 135.25,67.94 v135.25,74.93 v124.44,74.93
  Bottom 0.254: X4.37 v124.44,74.93
  Bottom 0.406: X5.37 X4.37 | U14.14 137.41,89.28 137.16,89.53 136.53,89.53 135.89,88.9 135.89,87 135.25,86.36 v135.25,74.93
PROG
  Top 0.406: R3.2 10.77,74.01 U1.5
RESET_DCHN
  Top 0.406: JP7.14 43.81,39.37 43.18,38.73 43.18,32.38 43.18,31.75 42.55,31.12 33.02,31.12 24.77,22.86 11.43,22.86 10.79,22.23 10.79,17.78 10.26,17.25 X6.8
RESET_IN  (via drill 0.6)
  Top 0.406: U15.3 17.78,45.72 17.14,45.09 12.7,45.09 v12.06,45.72
  Bottom 0.406: v12.06,45.72 10.16,47.62 10.16,50.8 10.16,52.07 10.06,52.17 X2.8
SCLK  (via drill 0.5, 0.6)
  Top 0.406: U2.1 57.38,52.3 v56.52,51.44 55.88,51.44 | U12.11 36.2,55.88 | 36.2,55.88 v36.83,55.88 | 55.88,51.44 55.25,50.8 55.25,46.99 53.97,45.72 53.97,34.29 55.25,33.02 55.25,30.48 54.61,29.84 54.61,28.58 55.25,27.94 55.25,26.67 55.25,24.77 55.88,24.13 57.15,24.13 57.38,23.9 U5.1 57.38,21.18 55.88,19.68 55.88,15.88 56.52,15.24 56.52,8.25 62.86,1.9 63.5,1.9 64.77,1.9 134.62,1.9 139.06,1.9 140.97,1.9 141.6,1.9 v146.05,6.35 | U7.1 143.92,21.36 v144.78,22.23 | U13.1 143.92,75.97 144.15,76.2 146.69,76.2 v147.32,76.84 | U10.1 143.92,49.94 144.15,50.16 146.05,50.16 v147.32,51.44 | v145.42,66.68 145.42,59.05 v145.42,57.78 | v142.88,40.01 142.88,39.37 143.51,38.73 143.51,37.46 142.88,36.83 142.88,35.56 143.51,34.92 144.78,33.66 v144.78,31.12 147.96,31.12 154.94,38.1 154.94,46.35 156.84,48.26 157.28,48.69 159.82,48.69 X3.2 | v36.83,55.88 36.2,55.88 | 53.97,72.39 53.97,69.22 53.97,68.58 53.97,67.94 53.97,56.52 53.34,55.88 53.34,53.98 53.97,53.34 54.61,52.7 55.88,51.44 | 53.97,72.39 53.97,74.29 53.97,74.93 v56.52,77.47 | v36.83,55.88 37.47,55.88 39.37,57.78 51.44,57.78 52.07,58.42 52.07,67.94 52.07,68.58 50.8,69.85 50.17,70.49 50.17,71.75 50.8,72.39 53.97,72.39
  Bottom 0.406: U6.1 57.38,44.22 55.88,45.72 55.88,50.8 v56.52,51.44 | U3.1 57.38,76.61 v56.52,77.47 | U14.1 143.92,80.87 144.15,80.65 145.42,79.38 146.69,79.38 147.32,78.74 v147.32,76.84 147.32,76.2 147.32,69.85 145.42,67.94 145.42,67.31 v145.42,66.68 | v145.42,57.78 143.92,56.92 U11.1 143.92,55.47 144.78,54.61 145.42,53.98 146.69,53.98 147.32,53.34 v147.32,51.44 142.88,46.99 v142.88,40.01 | v144.78,31.12 144.15,30.48 143.92,30.25 U9.1 143.92,27.53 144.15,27.3 145.42,27.3 147.32,25.4 147.32,23.5 146.05,22.23 v144.78,22.23 144.78,19.68 144.78,18.41 145.42,17.78 146.05,17.14 146.05,8.25 v146.05,6.35 | v36.83,55.88 38.1,54.61 38.1,50.16 38.1,47.62 40,45.72 40.64,45.09 40.64,43.81 41.91,42.55 JP7.11
SCLK_DCHN
  Top 0.406: JP7.12 45.09,41.91 | 45.09,41.91 | 45.09,41.91 45.72,41.27 45.72,31.12 45.09,30.48 33.66,30.48 25.4,22.23 14.61,22.23 13.97,22.23 13.33,21.59 13.33,20.95 13.33,15.88 13.33,13.97 12.5,13.13 10.59,13.13 X6.2
SCLK_IN
  Top 0.406: U12.6 16.51,55.88 12.07,51.44 12.06,51.44 10.79,50.16 10.79,48.9 9.96,48.06 X2.2
STAT  (via drill 0.6)
  Top 0.406: U1.1 14.29,76.52 14.61,76.2 v14.61,75.56 | v13.97,71.75 R1.1 R2.1
  Bottom 0.406: v14.61,75.56 14.61,74.93 14.61,72.39 v13.97,71.75
SW
  Top 0.406: U4.4 U4.3 29.21,81.05 29.21,81.28 28.57,81.91 28.57,90.17 28.4,90.34 L1.2
  pour Top (isolate 0.305, no thermals): 29.59,81.91 29.25,82.42 arc-34 29.21,82.56 29.21,91.44 27.94,91.44 27.94,82.63 arc36 27.99,82.48 28.83,81.34 28.83,80.45 29.59,80.45
SYNC_DCHN  (via drill 0.6)
  Top 0.406: JP7.6 45.72,49.53 | 45.72,49.53 v46.99,49.53 45.72,49.53
  Bottom 0.406: X6.4 10.16,18.62 13.54,18.62 14.61,19.68 15.24,20.32 27.3,20.32 34.92,27.94 35.56,28.58 46.99,28.58 47.62,29.21 47.62,29.84 47.62,40.64 46.99,41.27 46.99,41.91 46.99,46.35 46.36,46.99 46.36,48.9 v46.99,49.53
SYNC_IN
  Top 0.406: X2.4 10.36,53.54 16.51,59.69 U12.3
TEST_1  (via drill 0.6)
  Top 0.406: U15.12 33.66,43.18 34.29,43.81 34.61,44.13 R23.2 38.41,44.13 v38.73,43.81 38.73,52.07 38.73,53.34 38.73,53.98 38.73,54.61 40.64,56.52 51.44,56.52 52.07,55.88 52.07,40.64 50.17,38.73 50.17,19.68 50.8,19.05 52.07,17.78 v52.07,11.43
  Bottom 0.406: X3.5 161.52,57.78 161.93,57.78 163.2,57.78 163.83,57.78 165.1,56.52 165.1,55.88 165.1,46.99 162.56,44.45 161.29,44.45 | 161.29,44.45 160.66,44.45 | v52.07,11.43 62.86,0.63 63.5,0.63 64.14,0.63 134.62,0.63 146.69,0.63 154.94,8.89 154.94,36.2 156.21,37.46 156.21,40.64 156.21,41.91 158.75,44.45 161.29,44.45 | v38.73,43.81 38.73,43.18 38.73,42.55 40,41.27 40,38.73 40.64,38.1 40.64,37.46 41.27,36.83 JP7.15 | JP7.15
TEST_1_DCHN
  Bottom 0.406: JP7.16 45.09,36.83 45.72,36.2 45.72,32.38 45.72,31.12 45.09,30.48 33.66,30.48 32.38,29.21 25.4,22.23 9.75,22.23 X6.5
TEST_1_IN  (via drill 0.6)
  Top 0.406: v14.61,43.81 15.24,43.18 U15.5
  Bottom 0.406: v14.61,43.81 13.97,44.45 13.97,54.61 12.29,56.29 X2.5
TEST_2  (via drill 0.6)
  Top 0.406: U13.18 140,70.79 140.97,71.75 v141.6,72.39 | v145.42,74.29 146.05,74.29 | 146.05,74.29 146.69,74.29 148.59,76.2 148.59,80.01 145.42,83.19 142.88,83.19 142.24,83.82 141.92,84.14 | 141.92,84.14 141.6,84.46 | v141.6,89.53 141.6,84.46 | 141.6,84.46 141.92,84.14 | v157.48,51.44 155.58,53.34 155.58,60.32 155.58,64.77 153.67,66.68 153.67,69.85 153.67,71.12 150.5,74.29 146.05,74.29 | 29.21,41.91 33.34,41.91 R24.2 34.61,41.59 35.56,40.64 38.1,40.64 | 29.21,41.91 | 29.21,41.91 U15.11 | 38.1,40.64 v38.73,40.64 | v50.8,17.14 49.53,18.41 49.53,39.37 51.44,41.27 51.44,55.24 50.8,55.88 41.27,55.88 40.64,55.24 40.64,53.98 40.64,53.34 40.64,42.55 v38.73,40.64 | v38.73,40.64 38.1,40.64
  Bottom 0.406: v141.6,72.39 143.51,72.39 v145.42,74.29 | U14.18 140,89.2 140.34,89.53 v141.6,89.53 | v157.48,51.44 157.48,48.26 157.48,47.22 158.75,45.95 | 158.75,45.95 159.79,45.95 X3.1 | v50.8,17.14 51.44,17.14 53.34,15.24 53.34,11.43 63.5,1.27 64.14,1.27 134.62,1.27 145.42,1.27 153.67,9.53 153.67,36.83 153.67,37.46 153.67,40.87 154.31,41.5 158.75,45.95 | v38.73,40.64 38.73,36.83 40,35.56 40,34.92 40.64,34.29 JP7.17 | JP7.17
TEST_2_DCHN
  Bottom 0.406: X6.1 8.03,9.53 5.08,9.53 4.45,10.16 4.45,20.95 6.35,22.86 24.77,22.86 31.12,29.21 33.02,31.12 43.81,31.12 44.45,31.75 44.45,32.38 | JP7.18 44.45,32.38 | 44.45,32.38
TEST_2_IN
  Top 0.406: U15.6 12.29,41.91 X2.1
VBATT_A
  Top 0.406: JP3.2 13.06,83.46 JP2.1 13.37,83.16 U1.3 | 16.83,79.38 JP4.1 15.55,79.38 C2.1
  pour Top (isolate 0.305, no thermals): 13.33,83.19 17.14,80.65 17.21,78.55 16.13,78.55 12.7,78.61 12.7,83.19
VBATT_B  (via drill 0.6)
  Top 0.406: U4.11 30.17,75.89 v29.84,75.56 | L1.1 22.86,90.98 22.86,82.55 21.59,81.28 | 21.27,80.65 20.32,80.65 20.32,79.38 | 20.32,79.38 20.32,78.1 arc90 20.95,77.47 25.4,77.47 26.38,77.47 26.67,77.76 U4.8 27.3,77.22 v27.3,75.56 26.99,75.25 R4.2 24.45,73.66 R15.2 T1.E | JP4.2 20.32,79.38
  Bottom 0.406: v29.84,75.56 v27.3,75.56
  pour Top (isolate 0.305, no thermals): 21.59,90.81 21.59,80.65 24.77,80.65 24.77,81.28 22.97,82.47 arc-56 22.86,82.69 22.86,90.81
  pour Top (isolate 0.305, no thermals): 27.94,77.72 27.94,74.93 20.95,74.93 19.05,78.1 19.05,79.38 20.32,79.38 20.32,77.47 26.04,77.47 26.67,77.72
  pour Top (no thermals): 22.73,72.83 23.37,72.71 23.37,73.98 22.73,73.85
  pour Top (no thermals): 21.59,82.55 19.05,80.65 19.05,79.38 20.32,79.38 20.32,80.65 21.59,80.65
VDD  (via drill 0.5, 0.6)
  Top 0.254: U8.2 43.93,86.25 44.45,85.72 45.72,84.46 46.36,83.82 46.36,82.59 C15.+
  Top 0.406: v56.52,56.52 57.15,55.88 57.78,55.88 58.04,55.62 U2.2 58.04,50.1 C8.2 57.15,49.21 57.15,46.99 v57.15,46.35 | U5.2 58.04,19.94 57.78,19.68 57.78,18.09 C7.2 57.78,17.46 57.78,15.88 v57.78,13.97 | v57.78,13.97 57.78,13.34 | 57.78,13.34 57.78,8.25 63.5,2.54 64.77,2.54 | v57.78,13.97 57.78,13.34 | 144.15,23.5 143.26,22.61 U7.2 143.26,19.3 143.51,19.05 v146.05,19.05 | 144.15,23.5 144.15,24.45 C12.2 | v146.05,24.77 146.05,24.13 145.42,23.5 144.15,23.5 | 144.15,51.44 143.26,50.55 143.26,49.91 U10.2 143.26,47.24 143.51,46.99 144.15,46.99 147.32,46.99 147.95,46.36 R19.2 148.27,41.27 v149.86,41.27 | 144.15,51.44 144.15,52.39 C17.2 | 144.15,51.44 145.42,51.44 146.05,52.07 v146.05,52.7 | U13.2 143.26,76.58 143.51,76.84 144.15,76.84 | 144.15,76.84 144.15,77.79 C23.2 | 144.15,76.84 145.42,76.84 146.05,77.47 v146.05,78.1 146.05,80.65 144.78,81.91 142.88,81.91 140.34,84.46 140.34,90.17 v139.7,90.81 | R21.2 147.96,69.22 | 147.96,69.22 | 147.96,69.22 149.23,69.22 149.86,68.58 149.86,59.05 | 149.86,59.05 149.86,56.52 v146.05,52.7 | U13.17 139.37,67.64 139.7,67.31 141.6,67.31 142.24,66.68 v143.51,65.41 143.51,57.78 146.05,55.24 v146.05,52.7 | v149.86,10.16 149.55,9.84 R17.2 146.37,9.84 146.05,9.53 139.06,2.54 138.43,2.54 137.8,2.54 135.89,2.54 133.99,2.54 65.41,2.54 64.77,2.54 | C25.1 C24.1 30.8,49.21 | U12.16 29.84,62.23 30.8,63.18 C19.1 C18.1 35.88,63.18 v36.2,62.87 36.83,62.87 39.37,60.32 46.36,60.32 48.26,62.23 48.26,74.93 v51.44,78.1 51.44,80.01 48.86,82.59 46.36,82.59 | U15.16 29.84,48.26 30.8,49.21 | v151.13,59.05 149.86,59.05 | 30.8,49.21 35.88,49.21 v36.2,49.53
  Top 0.406: 64.14,2.54 64.77,2.54 | C17.2
  Bottom 0.406: U3.2 58.04,79.44 C6.2 | C6.2 | C6.2 53.34,80.01 v51.44,78.1 51.44,76.51 53.34,74.61 | R7.2 53.34,74.61 | 53.34,74.61 53.02,74.61 | v56.52,56.52 56.52,59.69 54.93,61.27 R6.2 54.61,66.68 56.52,68.58 56.52,69.85 55.25,71.12 53.34,71.12 53.34,71.75 53.34,74.61 | v57.78,13.97 57.15,14.61 55.88,15.88 55.88,19.05 55.25,19.68 53.34,21.59 53.34,23.5 53.97,24.13 54.93,24.13 R12.2 55.25,26.04 52.07,29.21 52.07,35.56 50.17,37.46 50.17,38.73 51.44,40.01 52.39,40.95 R13.2 53.65,40.64 57.78,40.64 58.04,40.9 U6.2 58.04,45.46 v57.15,46.35 57.15,49.21 C8.2 | U9.2 143.26,26.92 143.51,26.67 144.15,26.67 144.46,26.35 C13.2 | v146.05,24.77 C13.2 | C13.2 | v146.05,52.7 C17.2 | C17.2 | C23.2 v146.05,78.1 146.05,76.2 146.69,75.56 146.69,70.49 146.05,69.85 143.51,67.31 v143.51,65.41 146.05,65.41 146.69,66.04 146.69,66.68 147,66.99 R20.2 | C23.2 | U14.2 143.26,80.26 143.51,80.01 144.15,79.38 144.15,78.42 C23.2 | U11.2 143.26,54.86 143.51,54.61 144.15,53.98 144.15,53.02 C17.2 | R18.2 | U14.17 139.37,89.84 139.37,90.47 v139.7,90.81 142.24,90.81 142.56,90.49 R22.2 | R18.2 148.91,35.24 149.86,36.2 v149.86,41.27 | v149.86,10.16 149.86,10.79 | 149.86,10.79 149.86,11.43 149.86,13.34 149.86,14.61 149.86,33.34 R18.2 | v146.05,19.05 146.69,18.41 146.69,16.51 146.69,14.61 146.69,13.97 147.96,12.7 149.86,10.79 | X3.9 154.64,55.55 v151.13,59.05 | v36.2,49.53 35.56,50.16 34.29,51.44 34.29,60.96 34.29,62.23 34.92,62.87 v36.2,62.87 36.83,62.87 41.27,58.42 41.27,55.88 41.91,55.24 JP7.1 | C23.2 | C23.2
  pour Top (no thermals): 45.09,83.82 43.75,85.92 43.75,86.23 45.66,86.23 47.56,84.33 47.56,82.8 45.15,83.12 45.15,83.82
VDD_DCHN
  Bottom 0.406: X6.9 9.52,19.99 13.64,19.99 14.61,20.95 26.67,20.95 34.29,28.58 34.92,29.21 46.36,29.21 46.99,29.84 46.99,30.48 46.99,40.01 46.36,40.64 46.36,41.27 46.36,45.72 45.72,46.35 45.72,47.62 45.72,53.98 45.09,54.61 JP7.2
VREG  (via drill 0.4)
  Top 0.254: C11.1 38.73,86.68 | 38.73,86.68 39.75,86.68 U8.10 U8.11 | U8.8 39.17,87.75 38.73,86.68
  Top 0.406: U4.15 U4.16 | U4.16 31.84,80.74 U4.1 30.82,84.2 C10.+ 31.12,84.5 31.12,86.36 31.12,86.68 31.75,86.68 | R8.2 32.14,80.01 U4.16 | 31.75,86.68 C9.1 C11.1 | v31.75,87.63 31.75,86.68 | LED3.A 0.86,89.31 v1.27,88.9
  Bottom 0.406: v31.75,87.63 30.48,86.36 19.68,86.36 19.05,87 2.54,87 1.27,88.26 v1.27,88.9
  pour Top (isolate 0.305, no thermals): 30.73,80.39 31.5,80.39 31.5,78.99 33.91,78.99 33.91,81.28 33.66,81.28 33.66,88.26 30.48,88.26 30.48,81.91 30.73,81.91
VSET
  Top 0.406: U4.14 33.66,78.41 R10.2 34.3,77.79 34.36,77.73 R9.1
~RESET  (via drill 0.5, 0.6)
  Top 0.406: U5.23 58.04,30.23 57.78,30.48 v57.78,33.66 57.78,38.73 56.52,40.01 56.52,43.18 v55.88,43.81 | U2.23 58.04,63.24 57.78,63.5 57.78,65.41 v57.15,66.04 58.42,67.31 58.42,73.66 61.59,76.84 v61.59,79.38 | v149.23,71.75 144.78,71.75 143.51,71.75 143.26,71.5 U13.23 | U10.23 143.26,41.53 144.15,40.64 v144.15,36.2 144.15,35.56 144.78,34.92 146.05,34.92 146.69,35.56 149.86,35.56 151.77,37.46 v152.4,38.1 | U7.23 143.26,16.26 143.26,16.89 143.51,17.14 149.86,17.14 150.5,16.51 v152.4,16.51 | 141.6,1.27 134.62,1.27 64.77,1.27 62.86,1.27 62.23,1.27 55.25,8.25 55.25,15.24 55.25,18.41 52.7,20.95 v52.7,57.15 | 141.6,1.27 142.24,1.27 | v149.23,7.62 142.88,1.27 141.6,1.27 | v52.7,57.15 52.7,69.22 52.7,69.85 v51.44,71.12 | U15.14 34.92,45.72 36.83,45.72 37.47,46.35 37.47,50.16 36.83,50.8 v36.83,53.98 37.47,54.61 40,57.15 52.07,57.15 v52.7,57.15
  Bottom 0.406: v57.78,33.66 58.04,33.91 U6.23 | v57.15,66.04 57.15,66.68 58.04,67.56 U3.23 | 55.88,81.91 56.52,81.91 | 56.52,81.91 60.33,81.91 61.59,80.65 v61.59,79.38 | v55.88,43.81 52.7,46.99 v52.7,57.15 | U14.23 143.26,86.61 143.26,85.34 143.51,85.09 144.78,85.09 145.42,84.46 149.23,80.65 v149.23,71.75 149.23,69.85 150.5,68.58 150.5,64.77 149.23,63.5 143.51,63.5 143.26,63.25 U11.23 143.26,59.94 143.51,59.69 146.69,59.69 147.96,58.42 149.23,57.15 149.23,48.9 149.23,45.09 151.77,42.55 152.4,41.91 153.03,41.27 | U9.23 143.26,35.31 v144.15,36.2 | 153.03,41.27 153.03,38.73 v152.4,38.1 v152.4,16.51 152.4,10.79 v149.23,7.62 | X3.8 160.12,52.81 155.04,52.81 154.31,52.07 154.31,42.55 153.03,41.27 | v36.83,53.98 36.83,50.8 37.47,50.16 37.47,48.26 37.47,46.99 39.37,45.09 40,44.45 40,43.18 40.64,42.55 | 40.64,42.55 | v51.44,71.12 50.8,71.12 50.17,71.75 50.17,73.66 50.17,74.93 50.17,80.65 50.17,81.28 50.8,81.91 56.52,81.91 | 40.64,42.55 40.64,41.27 41.27,40.64 41.91,40.01 JP7.13 | JP7.13
~SYNC  (via drill 0.5, 0.6)
  Top 0.406: U2.24 57.38,60.73 v56.52,61.6 | U5.24 57.38,28.98 57.38,29.62 56.52,30.48 v56.52,34.29 55.88,34.92 55.88,41.91 v55.25,42.55 | U12.14 v35.56,59.69 36.2,59.69 48.26,59.69 48.89,60.32 v48.89,60.96 | v57.15,71.12 57.15,74.29 58.42,75.56 58.42,77.47 57.15,78.74 53.97,78.74 49.53,74.29 48.89,73.66 48.89,67.94 48.89,61.6 | U10.24 143.92,42.14 145.42,40.64 v145.42,36.2 148.59,36.2 152.4,40.01 153.03,40.64 v153.03,43.18 | U13.24 143.92,69.62 144.78,70.49 v150.5,70.49 | v148.59,15.88 147.96,15.88 144.15,15.88 143.92,15.65 U7.24 143.92,13.56 144.15,13.34 v144.78,13.34 | v48.89,60.96 48.89,61.6 | v48.89,60.96 48.89,61.6
  Bottom 0.406: v56.52,61.6 56.52,64.77 55.88,65.41 55.88,66.68 57.38,68.17 U3.24 57.38,70.26 57.38,70.89 v57.15,71.12 | v56.52,34.29 57.38,35.15 U6.24 | v55.25,42.55 52.07,45.72 51.44,46.35 | 143.92,87.22 U14.24 143.92,86.59 144.15,86.36 144.78,86.36 145.42,85.72 149.86,81.28 150.5,80.65 v150.5,70.49 151.77,69.22 151.77,63.5 151.13,62.87 144.15,62.87 143.92,62.64 U11.24 143.92,60.55 144.15,60.32 147.32,60.32 148.59,59.05 149.86,57.78 149.86,57.15 149.86,53.98 | U9.24 143.92,34.7 144.15,34.92 144.78,34.92 145.42,35.56 | 145.42,35.56 v145.42,36.2 | 149.86,53.98 149.86,46.35 v153.03,43.18 | v148.59,15.88 148.59,32.38 148.59,33.02 147.96,33.66 146.69,33.66 146.05,34.29 146.05,34.92 145.42,35.56 | v144.78,13.34 144.78,10.79 144.78,6.98 139.7,1.9 135.89,1.9 131.44,1.9 64.77,1.9 64.14,1.9 54.61,11.43 54.61,18.41 54.61,19.05 51.44,22.23 51.44,34.92 49.53,36.83 49.53,40.01 51.44,41.91 51.44,46.35 | X3.4 150.06,54.18 149.86,53.98 | v35.56,59.69 37.47,59.69 40,57.15 40,52.07 40,50.8 41.27,49.53 JP7.5 | JP7.5 | 51.44,46.35 51.44,52.07 51.44,56.52 49.53,58.42 48.89,59.05 v48.89,60.96
(copper drawn outside any net)
  shapes: Bottom area x1270

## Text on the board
Bottom: JIMMY 2015 / "THE ENABLER"
tPlace: PWR | + | LOW | CS IN | 33 | 34 | 35 | 36 | 37 | - | CHRG | SCOUSETOM V2.5 / SWITCH NETWORK | DAISY / CHAIN OUT | FULL | 8 | 7 | 6 | 5 | 4 | 3 | 2 | 1 | 25 | +5V | 26 | 27 | GND | 28 | 29 | SYNC | 30 | 31 | 32 | DIN+ | DIN- | SCLK | RST | ARDUINO / IN | TST1 | 16 | 15 | TST2 | 14 | 13 | 12 | 11 | 10 | DAISY / CHAIN / ON/OFF | 17 | 9 | 18 | 19 | 20 | 21 | 22 | 23 | 24 | DAISY / CHAIN IN | github.com/EIT-team/ScouseTom
bPlace: TO ELECTRODES | 20 | 21 | 22 | 23 | 24 | 25 | 26 | 27 | 28 | 29 | 30 | 31 | 33 | 34 | 35 | 36 | 37 | 32 | 10 | 11 | 12 | 13 | 14 | 15 | 16 | 17 | 18 | 19 | 1 | 2 | 3 | 4 | 5 | 6 | 7 | 8 | 9 | ARDUINO IN | DAISY CHAIN / OUT | TST1 | +5V | +5V | SYNC | GND | RST | SYNC | DIN+ | DIN- | SCLK | GND | DIN+ | DIN- | TST2 | SCLK | RST | TST1 | TST2 | TST1 | +5V | SYNC | RST | DIN+ | DIN- | SCLK | 10 | 11 | 12 | 13 | 14 | 15 | 16 | 17 | 18 | 19 | GND | 1 | 2 | 3 | 4 | 5 | 6 | 7 | 8 | 9 | TST2 | DAISY CHAIN / IN | 20 | 21 | 22 | 23 | 24 | 25 | 26 | 27 | 28 | 29 | 30 | 31 | 32 | 33 | 34 | 35 | 36 | 37 | TO EEG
